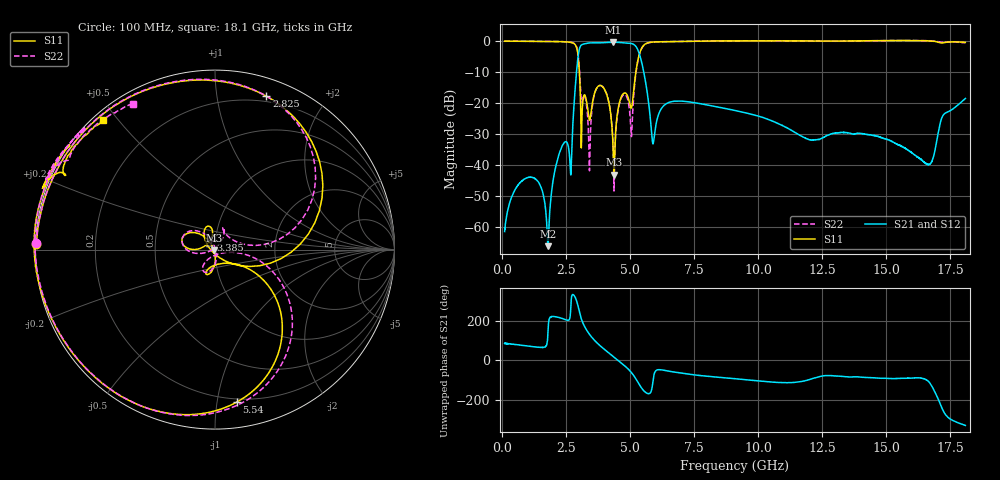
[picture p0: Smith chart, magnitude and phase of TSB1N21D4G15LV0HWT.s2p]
! TSB1N21D4G15LV0HWT  S-PARAMETER MODEL  ( General Type )
! Model Generated by TAIYO YUDEN Corporation (https://www.yuden.co.jp/en/)
! Version 1.0
! TAIYO YUDEN Control No. 20240527
! Copyright(c) 2024 TAIYO YUDEN CO.,LTD. All Rights Reserved.
! Products Name : Ceramic RF Devices
! Characteristics :
!  Passband freq : 3300-5000MHz ( At Passband , Insertion Loss : 1.3dB , VSWR  )
!  Attenuation : 27 dB min at 700 to 2690MHz, 17 dB min at 6000 to 8000MHz, Impedance : 50 Ohm
!  Case Size : 2 x 1.25 / 0.079 x 0.049 [mm/inch] , Thickness : 0.65/ 0.026 [mm/inch]
!  (Conditions: Temperature = 25 degC , DC Bias Current/Voltage = 0A / 0V)
! External Node Assignments :
!  1  o---|-------|---o  2
!  |  BPF  |
! GND o---|-------|---o GND
! Frequency Range : 100MHz  -  18.1GHz  [ 3601 STEP ]
# MHZ S RI R 50
! Freq[MHz].  S11 Real  S11 Imag  S21 Real  S21 Imag  S12 Real  S12 Imag  S22 Real  S22 Imag
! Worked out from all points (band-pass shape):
!   3601 points, 100 MHz to 18.1 GHz, reference 50 ohm
!   highest |S21| = -0.38 dB at 4.33 GHz (marker M1); lowest = -66.0 dB at 1.8 GHz (marker M2)
!   |S21| within 3 dB of the highest: 3.001 GHz to 5.332 GHz (2.331 GHz wide, 55.9 % of centre)
!   lowest |S11| = -43.0 dB at 4.375 GHz (marker M3), VSWR 1.01, Z = 49.4 - j0.347 ohm
!   |S11| at or under -10 dB: 3.02 GHz to 5.227 GHz (2.207 GHz wide, 53.5 % of centre)
!   |S22| runs from -48.3 to 0.2 dB; largest |S21 - S12| = 0.0022
!   S11 on the Smith chart (normalised r, x): 100 MHz: 0.00, +0.02; 2.825 GHz: 0.15, +1.38; 3.385 GHz: 0.95, +0.11; 5.54 GHz: 0.18, -1.14; 18.1 GHz: 0.03, +0.46
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100  -0.9952 0.0338  7.12e-05 0.000858  8.05e-05 0.000848  -0.9956 0.0347
1090  -0.9334 0.3282  0.00216 0.00611  0.00216 0.0061  -0.9302 0.3373
1800  -0.8079 0.5635  -0.000468 0.000176  -0.000472 0.00018  -0.8012 0.5748
2225  -0.6346 0.7467  -0.0121 -0.00899  -0.0121 -0.00892  -0.6277 0.7546
2675  -0.1253 0.9437  -0.00339 -0.00669  -0.00345 -0.00669  -0.1405 0.9465
2825  0.286 0.8549  0.095 -0.0637  0.095 -0.0638  0.2408 0.8792
3100  -0.0195 -0.0062  -0.7562 -0.4169  -0.7555 -0.4171  0.0885 0.061
3385  -0.0244 0.0553  -0.6784 0.6342  -0.6787 0.6336  0.0132 0.022
3885  -0.1735 0.0776  0.3584 0.8664  0.3576 0.8655  -0.171 0.0836
4330  -0.0147 0.0176  0.8967 0.3359  0.8959 0.3361  -0.00461 0.0239
4375  -0.00615 -0.00352  0.9206 0.2618  0.9202 0.2617  0.00364 0.00128
4675  -0.0241 -0.1288  0.9084 -0.2518  0.9083 -0.2514  -0.0303 -0.1219
5115  0.0968 -0.0775  0.2692 -0.8534  0.2699 -0.8524  0.0866 -0.0146
5540  0.1208 -0.8499  -0.2809 -0.1305  -0.2809 -0.1317  0.1898 -0.8311
5880  -0.4042 -0.8741  -0.0122 -0.0197  -0.0122 -0.0198  -0.3776 -0.8834
6100  -0.5822 -0.7791  0.0424 -0.0471  0.0424 -0.0471  -0.5753 -0.7823
9100  -1.007 0.0264  -0.00468 -0.0762  -0.00474 -0.0762  -0.9977 0.1348
12100  -0.8296 0.5615  -0.0018 -0.0254  -0.00184 -0.0255  -0.7404 0.6672
15100  -0.9358 0.3982  -0.001 -0.0256  -0.000933 -0.0257  -0.9106 0.4561
16695  -0.9305 0.386  -0.00395 -0.00964  -0.00408 -0.00961  -0.9109 0.4335
17225  -0.8373 0.4139  -0.0179 0.0608  -0.0174 0.0612  -0.812 0.5063
18100  -0.622 0.7209  0.1036 0.0588  0.1035 0.0586  -0.4595 0.812
